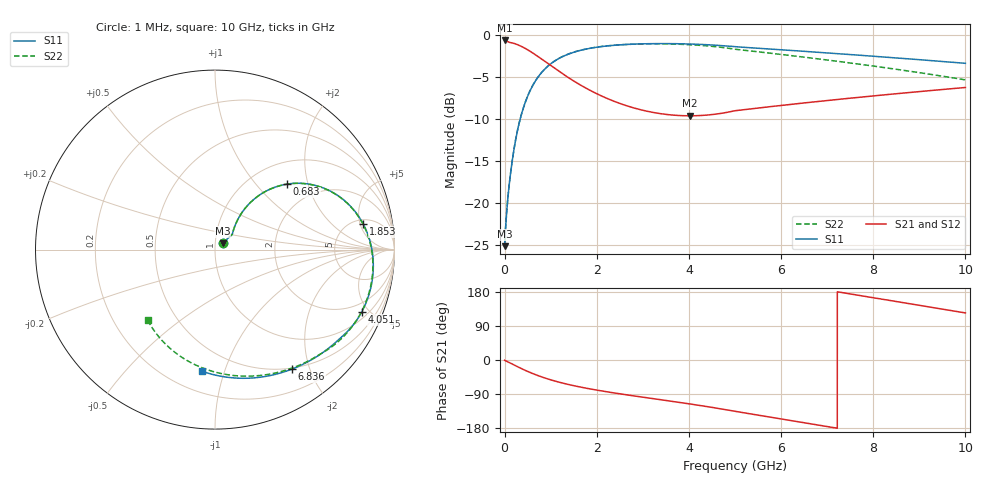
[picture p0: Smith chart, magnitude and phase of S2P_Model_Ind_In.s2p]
! Created Fri Jun 22 18:15:07 2018
# hz S ma R 50
! 2 Port Network Data from SP2.SP block
! freq  magS11  angS11  magS21  angS21  magS12  angS12  magS22  angS22
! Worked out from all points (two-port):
!   10000 points, 1 MHz to 10 GHz, reference 50 ohm
!   highest |S21| = -0.60 dB at 1 MHz (marker M1); lowest = -9.6 dB at 4.019 GHz (marker M2)
!   |S21| within 3 dB of the highest: start of sweep to 1.003 GHz
!   lowest |S11| = -25.1 dB at 1 MHz (marker M3), VSWR 1.12, Z = 54.2 + j3.91 ohm
!   |S11| at or under -10 dB: start of sweep to 337.8 MHz
!   |S22| runs from -25.1 to -1.0 dB; largest |S21 - S12| = 0
!   S11 on the Smith chart (normalised r, x): 1 MHz: 1.08, +0.08; 683 MHz: 1.44, +1.48; 1.853 GHz: 5.83, +5.62; 4.051 GHz: 1.37, -4.51; 6.836 GHz: 0.48, -1.73; 10 GHz: 0.33, -0.84
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1000000  0.0553 40.6  0.9331 -0.7  0.9331 -0.7  0.05528 40.6
1.23e8  0.1447 45.6  0.9072 -7.9  0.9072 -7.9  0.1448 45.6
1.91e8  0.1983 52.2  0.8983 -12.2  0.8983 -12.2  0.1984 52.2
2.65e8  0.2585 54.0  0.8841 -16.7  0.8841 -16.7  0.2587 54.0
4.47e8  0.3971 50.6  0.8372 -27.3  0.8372 -27.3  0.3974 50.5
6.83e8  0.5421 42.3  0.7622 -39.2  0.7622 -39.2  0.5426 42.2
8.96e8  0.6389 34.8  0.6933 -48.3  0.6933 -48.3  0.6395 34.7
1.158e9  0.7231 26.6  0.6166 -57.7  0.6166 -57.7  0.7238 26.4
1.668e9  0.8173 13.8  0.5019 -72.0  0.5019 -72.0  0.8182 13.4
1.853e9  0.8377 9.9  0.4706 -76.3  0.4706 -76.3  0.8385 9.4
2.532e9  0.8796 -2.2  0.3901 -89.8  0.3901 -89.8  0.8799 -3.3
3.334e9  0.8938 -13.8  0.343 -103.9  0.343 -103.9  0.8912 -16.3
4.019e9  0.8888 -22.6  0.3314 -115.9  0.3314 -115.9  0.8804 -27.1
4.051e9  0.8882 -23.0  0.3314 -116.5  0.3314 -116.5  0.8795 -27.7
5.001e9  0.856 -34.7  0.3554 -135.5  0.3554 -135.5  0.827 -44.5
5.831e9  0.8271 -44.9  0.3776 -152.1  0.3776 -152.1  0.7798 -59.4
6.667e9  0.7979 -55.2  0.3999 -168.9  0.3999 -168.9  0.7323 -74.3
6.836e9  0.792 -57.2  0.4044 -172.3  0.4044 -172.3  0.7227 -77.3
7.561e9  0.7668 -66.1  0.4238 173.2  0.4238 173.2  0.6815 -90.2
8.334e9  0.7398 -75.6  0.4445 157.7  0.4445 157.7  0.6376 -104.0
9.193e9  0.7099 -86.1  0.4674 140.4  0.4674 140.4  0.5888 -119.4
1e10  0.6817 -96.0  0.489 124.2  0.489 124.2  0.5429 -133.8
